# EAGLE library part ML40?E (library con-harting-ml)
HARTING
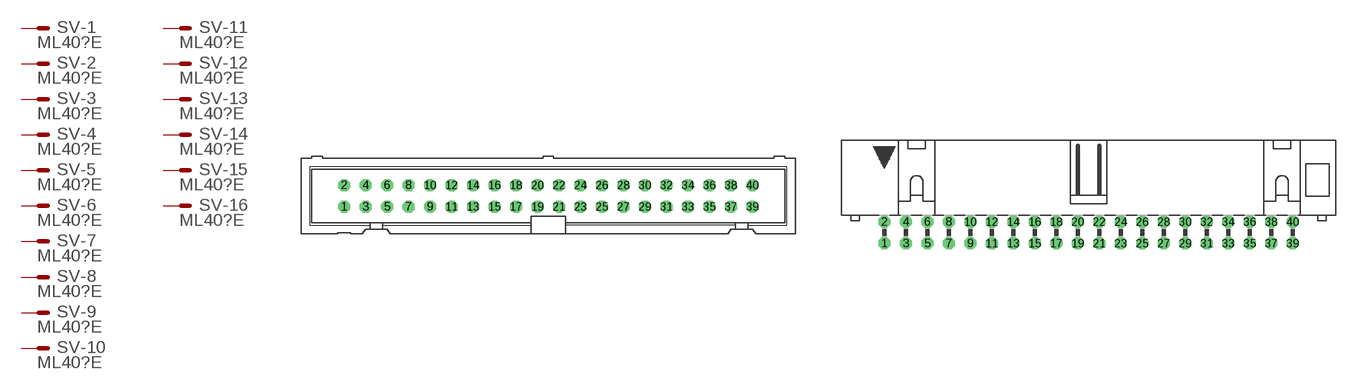
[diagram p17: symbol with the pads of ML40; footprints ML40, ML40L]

Designator prefix SV; gates -1=M -2=M -3=M -4=M -5=M -6=M -7=M -8=M -9=M -10=M -11=M -12=M -13=M -14=M -15=M -16=M -17=M -18=M -19=M -20=M -21=M -22=M -23=M -24=M -25=M -26=M -27=M -28=M -29=M -30=M -31=M -32=M -33=M -34=M -35=M -36=M -37=M -38=M -39=M -40=M

## ML40E (OC_FARNELL: unknown; OC_NEWARK: unknown)  [ML40]
1  -1:S  pas
2  -2:S  pas
3  -3:S  pas
4  -4:S  pas
5  -5:S  pas
6  -6:S  pas
7  -7:S  pas
8  -8:S  pas
9  -9:S  pas
10  -10:S  pas
11  -11:S  pas
12  -12:S  pas
13  -13:S  pas
14  -14:S  pas
15  -15:S  pas
16  -16:S  pas
17  -17:S  pas
18  -18:S  pas
19  -19:S  pas
20  -20:S  pas
21  -21:S  pas
22  -22:S  pas
23  -23:S  pas
24  -24:S  pas
25  -25:S  pas
26  -26:S  pas
27  -27:S  pas
28  -28:S  pas
29  -29:S  pas
30  -30:S  pas
31  -31:S  pas
32  -32:S  pas
33  -33:S  pas
34  -34:S  pas
35  -35:S  pas
36  -36:S  pas
37  -37:S  pas
38  -38:S  pas
39  -39:S  pas
40  -40:S  pas

## ML40LE (OC_FARNELL: unknown; OC_NEWARK: unknown)  [ML40L]
Pads as for ML40

## ML403ME (OC_FARNELL: unknown; OC_NEWARK: unknown)  [3M_40]
Pads as for ML40

## ML403MLE (OC_FARNELL: unknown; OC_NEWARK: unknown)  [3M_40L]
Pads as for ML40

## Footprint ML40 (pad centres in mm)
HARTING
drill 0.914 octagon: 1 -24.13,-1.27; 2 -24.13,1.27; 3 -21.59,-1.27; 4 -21.59,1.27; 5 -19.05,-1.27; 6 -19.05,1.27; 7 -16.51,-1.27; 8 -16.51,1.27; 9 -13.97,-1.27; 10 -13.97,1.27; 11 -11.43,-1.27; 12 -11.43,1.27; 13 -8.89,-1.27; 14 -8.89,1.27; 15 -6.35,-1.27; 16 -6.35,1.27; 17 -3.81,-1.27; 18 -3.81,1.27; 19 -1.27,-1.27; 20 -1.27,1.27; 21 1.27,-1.27; 22 1.27,1.27; 23 3.81,-1.27; 24 3.81,1.27; 25 6.35,-1.27; 26 6.35,1.27; 27 8.89,-1.27; 28 8.89,1.27; 29 11.43,-1.27; 30 11.43,1.27; 31 13.97,-1.27; 32 13.97,1.27; 33 16.51,-1.27; 34 16.51,1.27; 35 19.05,-1.27; 36 19.05,1.27; 37 21.59,-1.27; 38 21.59,1.27; 39 24.13,-1.27; 40 24.13,1.27

## Footprint ML40L (pad centres in mm)
HARTING
drill 0.914 octagon: 1 -24.13,-1.27; 2 -24.13,1.27; 3 -21.59,-1.27; 4 -21.59,1.27; 5 -19.05,-1.27; 6 -19.05,1.27; 7 -16.51,-1.27; 8 -16.51,1.27; 9 -13.97,-1.27; 10 -13.97,1.27; 11 -11.43,-1.27; 12 -11.43,1.27; 13 -8.89,-1.27; 14 -8.89,1.27; 15 -6.35,-1.27; 16 -6.35,1.27; 17 -3.81,-1.27; 18 -3.81,1.27; 19 -1.27,-1.27; 20 -1.27,1.27; 21 1.27,-1.27; 22 1.27,1.27; 23 3.81,-1.27; 24 3.81,1.27; 25 6.35,-1.27; 26 6.35,1.27; 27 8.89,-1.27; 28 8.89,1.27; 29 11.43,-1.27; 30 11.43,1.27; 31 13.97,-1.27; 32 13.97,1.27; 33 16.51,-1.27; 34 16.51,1.27; 35 19.05,-1.27; 36 19.05,1.27; 37 21.59,-1.27; 38 21.59,1.27; 39 24.13,-1.27; 40 24.13,1.27

## Footprint 3M_40 (pad centres in mm)
3M
drill 0.813 square: 1 -24.13,-1.27; 2 -24.13,1.27; 3 -21.59,-1.27; 4 -21.59,1.27; 5 -19.05,-1.27; 6 -19.05,1.27; 7 -16.51,-1.27; 8 -16.51,1.27; 9 -13.97,-1.27; 10 -13.97,1.27; 11 -11.43,-1.27; 12 -11.43,1.27; 13 -8.89,-1.27; 14 -8.89,1.27; 15 -6.35,-1.27; 16 -6.35,1.27; 17 -3.81,-1.27; 18 -3.81,1.27; 19 -1.27,-1.27; 20 -1.27,1.27; 21 1.27,-1.27; 22 1.27,1.27; 23 3.81,-1.27; 24 3.81,1.27; 25 6.35,-1.27; 26 6.35,1.27; 27 8.89,-1.27; 28 8.89,1.27; 29 11.43,-1.27; 30 11.43,1.27; 31 13.97,-1.27; 32 13.97,1.27; 33 16.51,-1.27; 34 16.51,1.27; 35 19.05,-1.27; 36 19.05,1.27; 37 21.59,-1.27; 38 21.59,1.27; 39 24.13,-1.27; 40 24.13,1.27

## Footprint 3M_40L (pad centres in mm)
3M
drill 0.813 square: 1 -24.13,-5.08; 2 -24.13,-2.54; 3 -21.59,-5.08; 4 -21.59,-2.54; 5 -19.05,-5.08; 6 -19.05,-2.54; 7 -16.51,-5.08; 8 -16.51,-2.54; 9 -13.97,-5.08; 10 -13.97,-2.54; 11 -11.43,-5.08; 12 -11.43,-2.54; 13 -8.89,-5.08; 14 -8.89,-2.54; 15 -6.35,-5.08; 16 -6.35,-2.54; 17 -3.81,-5.08; 18 -3.81,-2.54; 19 -1.27,-5.08; 20 -1.27,-2.54; 21 1.27,-5.08; 22 1.27,-2.54; 23 3.81,-5.08; 24 3.81,-2.54; 25 6.35,-5.08; 26 6.35,-2.54; 27 8.89,-5.08; 28 8.89,-2.54; 29 11.43,-5.08; 30 11.43,-2.54; 31 13.97,-5.08; 32 13.97,-2.54; 33 16.51,-5.08; 34 16.51,-2.54; 35 19.05,-5.08; 36 19.05,-2.54; 37 21.59,-5.08; 38 21.59,-2.54; 39 24.13,-5.08; 40 24.13,-2.54
hole 2.54 at -30.048,-3.277
hole 2.54 at 30.048,-3.277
